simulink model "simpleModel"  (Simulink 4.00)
settings: Solver=ode45  StartTime=0.0  StopTime=1000.0  RelTol=1e-3
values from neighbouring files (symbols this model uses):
  N = 360000    [blasterCodeRedCompare.m]    (also in KalmanDetection.m)
undefined symbols (not defined in the file or in its folder): beta, I_0
libraries: simulink3 x1

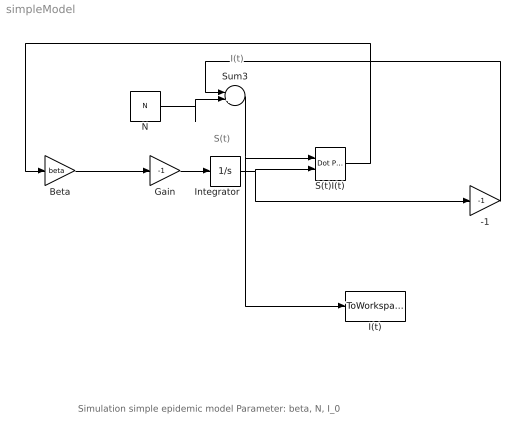
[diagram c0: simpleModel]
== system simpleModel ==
  note: S(t)
  note: I(t)
  note: Simulation simple epidemic model Parameter: beta, N, I_0
  -1 : Gain  Gain=-1  Multiplication=Element-wise(K.*u)  SaturateOnIntegerOverflow=on
  Beta : Gain  Gain=beta  Multiplication=Element-wise(K.*u)  SaturateOnIntegerOverflow=on
  Gain : Gain  Gain=-1  Multiplication=Element-wise(K.*u)  SaturateOnIntegerOverflow=on
  I(t) : ToWorkspace  VariableName=I_t  SampleTime=1  SaveFormat=Array
  Integrator : Integrator  ExternalReset=none  InitialConditionSource=internal  InitialCondition=N-I_0  LimitOutput=off  UpperSaturationLimit=inf  LowerSaturationLimit=-inf  ShowSaturationPort=off  ShowStatePort=off  AbsoluteTolerance=auto
  N : Constant  Value=N  VectorParams1D=off
  S(t)I(t) : simulink3/Math/Dot Product
  Sum3 : Sum  Inputs=|++  SaturateOnIntegerOverflow=on
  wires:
  Integrator/1 -> S(t)I(t)/2, -1/1
  Gain/1 -> Integrator/1
  Beta/1 -> Gain/1
  Sum3/1 -> S(t)I(t)/1, I(t)/1
  S(t)I(t)/1 -> Beta/1
  -1/1 -> Sum3/1
  N/1 -> Sum3/2
